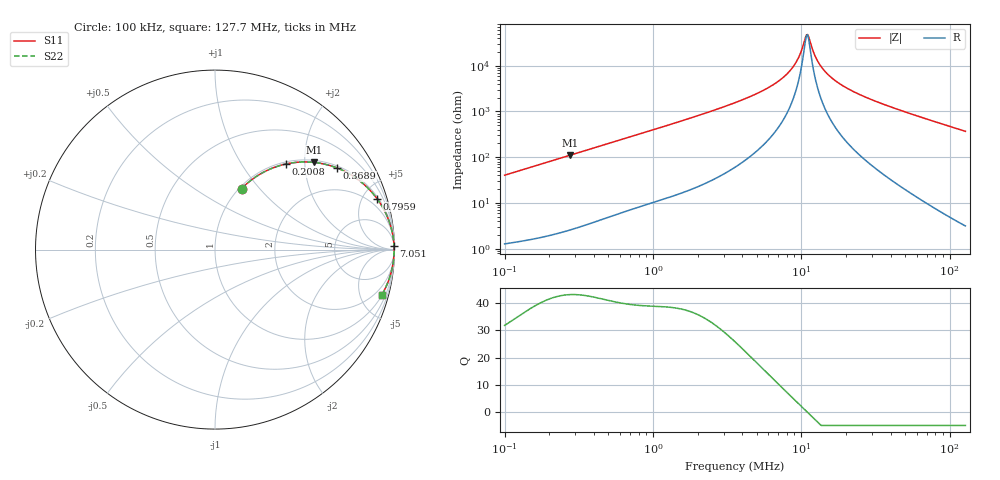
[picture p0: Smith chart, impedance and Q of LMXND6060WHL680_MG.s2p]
! LMXND6060WHL680_MG  S-PARAMETER MODEL  ( General Type )
! Model Generated by TAIYO YUDEN Corporation (http://www.ty-top.com)
! Version 1.0
! TAIYO YUDEN Control No. 191025NI43SB-FBB
! Copyright(c) 2019 TAIYO YUDEN CO.,LTD. All Rights Reserved.
! Product Description (link to TY-COMPAS)
! https://ds.yuden.co.jp/TYCOMPAS/or/detail?pn=LMXND6060WHL680MMG&u=M
! Products Name : Inductors
! Characteristics :
!  Inductance : 68 uH , SRF(min) : 5.0 MHz , DC Resistance(max) : 0.546 Ohm
!  Rated Current : Saturation :800 mA , Temp Rise : 770 mA
!  Case Size : 6.0 x 6.0 / 0.236 x 0.236 [mm/inch] , Thickness : 2.8 / 0.11 [mm/inch]
!  (Conditions: Temperature = 25 degC , DC Bias Current/Voltage = 0A / 0V)
! External Node Assignments :
!  1  o---GGG---o  2
! GND o---------o GND
! Frequency Range : 0.1MHz  -  127.746476MHz  [ 402 STEP ]
# MHz S RI R 50
! Freq[MHz].  S11 Real  S11 Imag  S21 Real  S21 Imag  S12 Real  S12 Imag  S22 Real  S22 Imag
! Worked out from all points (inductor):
!   401 points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, 100 kHz to 127.7 MHz, reference 50 ohm
!   read as one part in series: L = 64 uH near 103.6 kHz
!   highest Q = 43.2 at 277.1 kHz (marker M1), where L = 63.6 uH
!   self-resonance near 10.83 MHz
!   S11 on the Smith chart (normalised r, x): 100 kHz: 1.03, +0.81; 200.8 kHz: 1.04, +1.61; 368.9 kHz: 1.07, +2.94; 795.9 kHz: 1.16, +6.30; 7.051 MHz: 10, +93; 127.7 MHz: 1.06, -7.36
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0.1  0.1478 0.3395  0.8522 -0.3395  0.8522 -0.3395  0.1478 0.3395
0.200849  0.3956 0.4771  0.6044 -0.4771  0.6044 -0.4771  0.3956 0.4771
0.277112  0.5499 0.4861  0.4501 -0.4861  0.4501 -0.4861  0.5499 0.4861
0.33137  0.6333 0.4704  0.3667 -0.4704  0.3667 -0.4704  0.6333 0.4704
0.3689  0.6801 0.4549  0.3199 -0.4549  0.3199 -0.4549  0.6801 0.4549
0.795868  0.9026 0.284  0.0974 -0.284  0.0974 -0.284  0.9026 0.284
1.098062  0.9448 0.2159  0.0552 -0.2159  0.0552 -0.2159  0.9448 0.2159
3.574164  0.9934 0.0637  0.00657 -0.0637  0.00657 -0.0637  0.9934 0.0637
5.296923  0.9964 0.037  0.00359 -0.037  0.00359 -0.037  0.9964 0.037
7.051437  0.9974 0.0213  0.00258 -0.0213  0.00258 -0.0213  0.9974 0.0213
8.135881  0.9977 0.0141  0.00229 -0.0141  0.00229 -0.0141  0.9977 0.0141
9.057322  0.9978 0.00897  0.00215 -0.00897  0.00215 -0.00897  0.9978 0.00897
9.72889  0.9979 0.00559  0.00209 -0.00559  0.00209 -0.00559  0.9979 0.00559
10.83075  0.998 0.000557  0.00205 -0.000557  0.00205 -0.000557  0.998 0.000557
11.2251  0.998 -0.00112  0.00205 0.00112  0.00205 0.00112  0.998 -0.00112
11.84371  0.9979 -0.00363  0.00205 0.00363  0.00205 0.00363  0.9979 -0.00363
12.72188  0.9979 -0.007  0.00208 0.007  0.00208 0.007  0.9979 -0.007
13.66517  0.9979 -0.0104  0.00214 0.0104  0.00214 0.0104  0.9979 -0.0104
16.93579  0.9975 -0.021  0.00246 0.021  0.00246 0.021  0.9975 -0.021
23.78795  0.9964 -0.0399  0.00361 0.0399  0.00361 0.0399  0.9964 -0.0399
39.24654  0.992 -0.0768  0.00796 0.0768  0.00796 0.0768  0.992 -0.0768
127.7465  0.9294 -0.2519  0.0706 0.2519  0.0706 0.2519  0.9294 -0.2519
